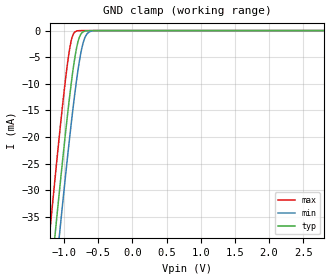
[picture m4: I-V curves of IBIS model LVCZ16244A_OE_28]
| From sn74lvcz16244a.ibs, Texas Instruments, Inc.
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[Model]   LVCZ16244A_OE_28
Model_type  Input
Vinl=0.8
Vinh=2
| variable   typ   min   max
C_comp   3.84pF   2.96pF   4.90pF
[Temperature Range]   40   100   -40
| Ambient temperature   25   85   -40
[Voltage range]   2.8   2.7   2.9
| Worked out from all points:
|   GND clamp passes 1 mA (typ) near -0.77 V on its own axis
[GND Clamp]
| LVCZ16244A_OE_28
|   Voltage   I(typ)   I(min)   I(max)
-5V       -583.8mA   -590.8mA   -575.1mA
-1.205V   -48.27mA   -56.56mA   -37.63mA
-1.13V    -38.42mA   -46.71mA   -27.77mA
-1.07V    -30.71mA   -38.96mA   -20.13mA
-1.05V    -28.19mA   -36.42mA   -17.65mA
-955mV    -16.68mA   -24.66mA   -6.874mA
-885mV    -9.098mA   -16.55mA   -1.486mA
-830mV    -4.281mA   -10.75mA   -171.6uA
-780mV    -1.472mA   -6.227mA   -17.15uA
-710mV    -173.7uA   -1.918mA   -639nA
-645mV    -18.49uA   -387.7uA   -29.98nA
2.8V      5.309pA    8.079pA    5.035pA
